TYPE stMisMotor :
STRUCT
	uiStatus AT %I* : UINT;				//Object 604!
	diActualpos AT %I* : DINT; 			//Position in motor counts

	uiCtrWord AT %Q* : UINT; 			//CANopen object 6040
	siModesOfOperation AT %Q*: SINT; 	//CANopen object 6060
	siModesOfOperationDisplay AT %I*: SINT; 	//CANopen object 6061
 
	diTargetpos AT %Q* : DINT; 			//Target pos in Counts
	diTargetVel AT %Q* : DINT;			//Target velocity in RPM/100 No direction 
	udiProfileVel AT %Q* : UDINT;		//Profile velocity in RPM/100 Direction input
	udiTargetAccel AT %Q* : UDINT; 		//Target accleration int RPM/sec

	State : eDSP402States; 				//CANopen FSA state		
	
	bEnableMotor : BOOL; 				//Start enable of the motor
	bQuickStop : BOOL ; 				//Set motor to quickstop mode
	
	wNodeId : WORD; 					//CANopen node id 
	ADSNetID : STRING(23); 				//ADS ID of can adapter. See system setting. Used for SDO communication
	lrUnitConversion : LREAL := 1.0 ; 	//Factor to convert from units to counts
	diRpmConversion : UDINT := 100; 	//Default conversion from RPM to motor velocity
	lrActualUnitPos : LREAL; 				//Position in converted units
END_STRUCT
END_TYPE
